FUNCTION_BLOCK FB_IEDClient IMPLEMENTS I_ScsmAbortIndEventSink, I_ScsmGetServerDirectoryCnfEventSink, I_ScsmGetLogicalDeviceDirectoryCnfEventSink, I_ScsmGetLogicalNodeDirectoryCnfEventSink, I_ScsmGetDataValuesCnfEventSink, I_ScsmSetDataValuesCnfEventSink, I_ScsmReportIndEventSink, I_ScsmControlCnfEventSink, I_ScsmLastApplErrorIndEventSink, I_ScsmCommandTerminationIndEventSink,
I_ScsmGetDataSetDirectoryCnfEventSink, I_ScsmCreateDataSetCnfEventSink, I_ScsmDeleteDataSetCnfEventSink
VAR_INPUT
	fbConnection		: FB_iec61850ClientClass := (ipAbortInd:=THIS^, ipGetServerDirectoryCnf:=THIS^, ipGetLogicalDeviceDirectoryCnf:=THIS^, ipGetLogicalNodeDirectoryCnf:=THIS^, ipGetDataValuesCnf:=THIS^, ipSetDataValuesCnf:=THIS^, ipReportInd:=THIS^, ipControlCnf:=THIS^, ipLastApplErrorInd:=THIS^, ipCommandTerminationInd:=THIS^,
													ipGetDataSetDirectoryCnf:=THIS^, ipCreateDataSetCnf:=THIS^, ipDeleteDataSetCnf:=THIS^);
END_VAR
VAR
	_bAbort				: BOOL; (* Rising edge activates AbortReq() command execution *)
	_bDisconnect		: BOOL; (* Rising edge activates ReleaseReq() command execution *)
	_bConnect			: BOOL; (* Rising edge activates AssociateReq() command execution *)
	_bReconnect			: BOOL := TRUE; (* TRUE => reconnect automatically *)
	_bReadAllData		: BOOL := TRUE; (* TRUE => read/refresh all data values on reconnect *)
	
	state				: BYTE;
	eState				: E_AsyncEnvironmentState; (* Environment state *)
	bBusy				: BOOL; (* If TRUE => command execution is busy *)
	bSuccess			: BOOL;
	ipResult			: I_AsyncServiceResultClass;
	sLastErrorResult	: T_MaxString;
	fbAbortReason		: FB_ServiceErrorClass := (stError:=SUCCESS_EVENT);
	sLastAbortReason	: T_MaxString;
	nInvokeID			: UDINT;
	eServiceError		: E_AcsiServiceError; (* Latest OnXyzCnf() or OnXyzInd() event handler error *)
	nServiceError		: UDINT; (* Counts OnXyzCnf() and OnXyzInd() event handler errors *)
	nCmdError			: UDINT; (* Counts xyzReq() command errors *)
	sObjReference		: T_AcsiObjectReference; (* DATA object reference *)
	sCtrlReference		: T_AcsiObjectReference; (* CONTROLLABLE-DATA object reference *)
	
	bGetServerDirectory				: BOOL := TRUE; (* Rising edge enumerates logical-devices *)
	bGetLogicalDeviceDirectory		: BOOL := TRUE; (* Rising edge enumerates logical-nodes *)
	bGetLogicalNodeDirectory		: BOOL := TRUE; (* Rising edge enumerates "IEDLD1/LLN0" data-sets *)
	bGetAllServerValues				: BOOL := TRUE; (* Rising edge reads all "IEDLD1" data attribute values *)
	bGetAllDataValues_LLN0_ST		: BOOL := TRUE; (* Rising edge reads all "IEDLD1/LLN0.ST" data attribute values (having selected functional constraint) *)
	bGetDataValues_LLN0_ST_Beh		: BOOL := TRUE; (* Rising edge reads all "IEDLD1/LLN0.ST.Beh" data attribute values (having selected functional constraint) *)
	
	bCreateDataSet_NonPersistent	: BOOL; (* Rising edge creates non-persistent data-set *)
	bCreateDataSet_Persistent		: BOOL; (* Rising edge creates persistent data-set *)
	
	bDeleteDataSet_NonPersistent	: BOOL; (* Rising edge deletes non-persistent data-set *)
	bDeleteDataSet_Persistent		: BOOL; (* Rising edge deletes persistent data-set *)
	
	bEnable_urcb101_NonPersistent	: BOOL; (* Rising edge enables urcb101 to report non-persistent data-set *)
	bEnable_urcb101_Persistent		: BOOL; (* Rising edge enables urcb101 to report persistent data-set *)
	bEnable_urcb101_DS1				: BOOL; (* Rising edge enables urcb101 to report static data-set *)
	bDisable_urcb101				: BOOL; (* Rising edge disables urcb101 reporting *)
	bSetDataValues_urcb101_DatSet	: BOOL; (* Rising edge writes empty string to "IEDLD1/LLN0.RP.urcb101.DatSet" attribute value *)

	bGetDataSetDirectory_NonPersistent : BOOL;(* Rising edge enumerates member of non-persistent data-set *)
	bGetDataSetDirectory_Persistent	: BOOL;(* Risign edge enumerates member of persistent data-set *)
	bGetDataSetDirectory_DS1		: BOOL;(* Rising edge enumerates member of static data-set *)
	
	(* If non-persistent or persistent data-set is used by any control-block then it is not possible 
		to delete it => Disable reporting and reconfigure the control-block to use an other data-set. *)
	
	fbNonPersistent					: FB_AcsiCommonDataSetClass:=(sObjectName:='NonPersistentDataSet');
	fbPersistent					: FB_AcsiCommonDataSetClass:=(sObjectName:='PersistentDataSet');
END_VAR

fbConnection.Execute();
eState:= fbConnection.eState;

CASE state OF
	0: (* Initial state *)
		IF _bAbort THEN (* Abort connection => execute AbortReq() command *)
			_bAbort:= FALSE;
			bSuccess:= fbConnection.AbortReq(ipReason:=fbAbortReason, ipSink:=0, ipResult=>ipResult);
			state:= SEL(bSuccess, 100, 1);
		ELSIF eState = E_AsyncEnvironmentState.Idle AND (_bConnect OR _bReconnect) THEN (* Open/establish connection => execute AssociateReq() command *)
			_bConnect:= FALSE;
			bGetAllServerValues:= SEL(_bReadAllData, bGetAllServerValues, TRUE);
			bSuccess:= fbConnection.AssociateReq(ipSink:=0, ipResult=>ipResult);
			state:= SEL(bSuccess, 100, 1);
		ELSIF eState = E_AsyncEnvironmentState.Established AND _bDisconnect THEN (* Close/release connection => execute ReleaseReq() command *)
			_bDisconnect:= FALSE;
			bSuccess:= fbConnection.ReleaseReq(ipSink:=0, ipResult=>ipResult);
			state:= SEL(bSuccess, 100, 1);
		ELSIF eState = E_AsyncEnvironmentState.Established THEN (* Connection established => exchange IED data *)
			state:= 10;
		END_IF
		_bConnect:= FALSE;
		_bDisconnect:= FALSE;
		(*==================================================================================================================================================================*)
	1: (* Wait for AbortReq() or ReleaseReq() or AssociateReq() command completion *)
		IF ipResult <> 0 THEN
			ipResult.Execute();
			IF NOT (bBusy:=ipResult.IsBusy()) THEN
				state:= SEL(ipResult.IsCompleted(), 100(* failed or aborted *), 0(* succeeded *));
			END_IF
		END_IF
		(*==================================================================================================================================================================*)
	10: (* Read/Write IED data *)
		IF bGetServerDirectory THEN (* Example => execute GetServerDirectoryReq() command *)
			bGetServerDirectory:= FALSE;
			bSuccess:= fbConnection.GetServerDirectoryReq(ipServer:=fbIED, eClass:=E_AcsiServerDirectoryClass.LogicalDevice, hUser:=0, ipSink:=0, nInvokeID=>nInvokeID, ipResult=>ipResult);
			state:= SEL(bSuccess, 100, 11);
		ELSIF bGetLogicalDeviceDirectory THEN (* Example => execute GetLogicalDeviceDirectoryReq() command *)
			bGetLogicalDeviceDirectory:= FALSE;
			bSuccess:= fbConnection.GetLogicalDeviceDirectoryReq(ipLogicalDevice:=fbIED.IEDLD1, hUser:=0, ipSink:=0, nInvokeID=>nInvokeID, ipResult=>ipResult);
			state:= SEL(bSuccess, 100, 11);
		ELSIF bGetLogicalNodeDirectory THEN (* Example => execute GetLogicalNodeDirectoryReq() command *)
			bGetLogicalNodeDirectory:= FALSE;
			bSuccess:= fbConnection.GetLogicalNodeDirectoryReq(ipLogicalNode:=fbIED.IEDLD1.LLN0, eClass:=E_AcsiLogicalNodeClass.DataSet, hUser:=0, ipSink:=0, nInvokeID=>nInvokeID, ipResult=>ipResult);
			state:= SEL(bSuccess, 100, 11);
		ELSIF bGetAllServerValues THEN (* Example => execute GetAllServerValues() command *)
			bGetAllServerValues:= FALSE;
			bSuccess:= fbConnection.GetAllServerValuesReq(ipServer:=fbIED, hUser:=0, ipSink:=0, nInvokeID=>nInvokeID, ipResult=>ipResult);
			state:= SEL(bSuccess, 100, 11);
		ELSIF bGetAllDataValues_LLN0_ST THEN (* Example => execute GetAllDataValuesReq() command *)
			bGetAllDataValues_LLN0_ST:= FALSE;
			bSuccess:= fbConnection.GetAllDataValuesReq(ipLogicalNode:=fbIED.IEDLD1.LLN0, eFc:=E_AcsiFc.ST_, hUser:=0, ipSink:=0, nInvokeID=>nInvokeID, ipResult=>ipResult);
			state:= SEL(bSuccess, 100, 11);
		ELSIF bGetDataValues_LLN0_ST_Beh THEN (* Example => execute GetDataValuesReq() command *)
			bGetDataValues_LLN0_ST_Beh:= FALSE;
			bSuccess:= fbConnection.GetDataValuesReq(ipData:=fbIED.IEDLD1.LLN0.Beh, eFc:=E_AcsiFc.ST_, hUser:=0, ipSink:=0, nInvokeID=>nInvokeID, ipResult=>ipResult);
			state:= SEL(bSuccess, 100, 11);
		(*==================================================================================================================================================================*)
		ELSIF bCreateDataSet_NonPersistent THEN (* Example => execute CreateDataSet(non-persistent) command *)
			bCreateDataSet_NonPersistent:= FALSE;
			IF fbNonPersistent.nMembers = 0 THEN (* Add some members *)
				bSuccess:= fbNonPersistent.AddMember(ipData:=fbIED.IEDLD1.XCBR1.Pos.stVal, eFc:=E_AcsiFc.ST_);
				bSuccess:= fbNonPersistent.AddMember(ipData:=fbIED.IEDLD1.LLN0.Mod_.stVal, eFc:=E_AcsiFc.ST_);
			END_IF
			bSuccess:= fbConnection.CreateDataSetReq(ipDataSet:=fbNonPersistent, ipLogicalNode:=0(* ipLogicalNode = 0 => non-persistent data-set *), hUser:=0, ipSink:=0, nInvokeID=>nInvokeID, ipResult=>ipResult);
			state:= SEL(bSuccess, 100, 11);
		(*==================================================================================================================================================================*)
		ELSIF bCreateDataSet_Persistent THEN (* Example => execute CreateDataSet(persistent) command *)
			bCreateDataSet_Persistent:= FALSE;
			IF fbPersistent.nMembers = 0 THEN (* Add some members *)
				bSuccess:= fbPersistent.AddMember(ipData:=fbIED.IEDLD1.MMXU1.TotW.mag.f, eFc:=E_AcsiFc.MX);
				bSuccess:= fbPersistent.AddMember(ipData:=fbIED.IEDLD1.LLN0.Beh.stVal, eFc:=E_AcsiFc.ST_);
			END_IF
			bSuccess:= fbConnection.CreateDataSetReq(ipDataSet:=fbPersistent, ipLogicalNode:=fbIED.IEDLD1.LLN0 (* ipLogicalNode <> 0 => persistent data-set *), hUser:=0, ipSink:=0, nInvokeID=>nInvokeID, ipResult=>ipResult);
			state:= SEL(bSuccess, 100, 11);
		(*==================================================================================================================================================================*)
		ELSIF bDeleteDataSet_NonPersistent THEN (* Example => execute DeleteDataSet(non-persistent) command *)
			bDeleteDataSet_NonPersistent:= FALSE;
			bSuccess:= fbConnection.DeleteDataSetReq(ipDataSet:=fbNonPersistent, hUser:=0, ipSink:=0, nInvokeID=>nInvokeID, ipResult=>ipResult);
			state:= SEL(bSuccess, 100, 11);
		(*==================================================================================================================================================================*)
		ELSIF bDeleteDataSet_Persistent THEN (* Example => execute DeleteDataSet(persistent) command *)
			bDeleteDataSEt_Persistent:= FALSE;
			bSuccess:= fbConnection.DeleteDataSetReq(ipDataSet:=fbPersistent, hUser:=0, ipSink:=0, nInvokeID=>nInvokeID, ipResult=>ipResult);
			state:= SEL(bSuccess, 100, 11);
		(*==================================================================================================================================================================*)
		ELSIF bEnable_urcb101_NonPersistent THEN (* Example => Enable urcb101 to use dynamic created non-persistent data-set *)
			bEnable_urcb101_NonPersistent:= FALSE;
			bSuccess:= fbIED.IEDLD1.LLN0.urcb101.Client.EnableReq(ipClient:=fbConnection, ipDataSet:=fbNonPersistent, ipResult=>ipResult);
			state:= SEL(bSuccess, 100, 11);
		(*==================================================================================================================================================================*)
		ELSIF bEnable_urcb101_Persistent THEN (* Example => Enable urcb101 to use dynamic created persistent data-set *)
			bEnable_urcb101_Persistent:= FALSE;
			bSuccess:= fbIED.IEDLD1.LLN0.urcb101.Client.EnableReq(ipClient:=fbConnection, ipDataSet:=fbPersistent, ipResult=>ipResult);
			state:= SEL(bSuccess, 100, 11);
		(*==================================================================================================================================================================*)
		ELSIF bEnable_urcb101_DS1 THEN (* Example => Enable urcb101 to use static data-set *)
			bEnable_urcb101_DS1:= FALSE;
			bSuccess:= fbIED.IEDLD1.LLN0.urcb101.Client.EnableReq(ipClient:=fbConnection, ipDataSet:=fbIED.IEDLD1.LLN0.DS1, ipResult=>ipResult);
			state:= SEL(bSuccess, 100, 11);
		(*==================================================================================================================================================================*)
		ELSIF bDisable_urcb101 THEN (* Example => Disable urcb101 *)
			bDisable_urcb101:= FALSE;
			bSuccess:= fbIED.IEDLD1.LLN0.urcb101.Client.DisableReq(ipResult=>ipResult);
			state:= SEL(bSuccess, 100, 11);
		(*==================================================================================================================================================================*)
		ELSIF bSetDataValues_urcb101_DatSet THEN(* Example => Set "DatSet" attribute value to empty string *)
			bSetDataValues_urcb101_DatSet:= FALSE;
			fbIED.IEDLD1.LLN0.urcb101.DatSet.sValue:= '';(* Set local "DatSet" attribute value to empty string *)
			(* Activate method to set the remote "DatSet" attribute value to empty string *)
			bSuccess:= fbConnection.SetDataValuesReq(ipData:=fbIED.IEDLD1.LLN0.urcb101.DatSet, eFc:=E_AcsiFc.RP, hUser:=0, ipSink:=0, nInvokeID=>nInvokeID, ipResult=>ipResult);
			state:= SEL(bSuccess, 100, 11);
		(*==================================================================================================================================================================*)
		ELSIF bGetDataSetDirectory_NonPersistent THEN (* Example => Enumerate member of non-persistent data-set *)
			bGetDataSetDirectory_NonPersistent:= FALSE;
			bSuccess:= fbConnection.GetDataSetDirectoryReq(ipDataSet:=fbNonPersistent, hUser:=0, ipSink:=0, nInvokeID=>nInvokeID, ipResult=>ipResult);
			state:= SEL(bSuccess, 100, 11);
		(*==================================================================================================================================================================*)
		ELSIF bGetDataSetDirectory_Persistent THEN (* Example => Enumerate member of persistent data-set *)
			bGetDataSetDirectory_Persistent:= FALSE;
			bSuccess:= fbConnection.GetDataSetDirectoryReq(ipDataSet:=fbPersistent, hUser:=0, ipSink:=0, nInvokeID=>nInvokeID, ipResult=>ipResult);
			state:= SEL(bSuccess, 100, 11);
		(*==================================================================================================================================================================*)
		ELSIF bGetDataSetDirectory_DS1 THEN (* Example => Enumerate member of static data-set *)
			bGetDataSetDirectory_DS1:= FALSE;
			bSuccess:= fbConnection.GetDataSetDirectoryReq(ipDataSet:=fbIED.IEDLD1.LLN0.DS1, hUser:=0, ipSink:=0, nInvokeID=>nInvokeID, ipResult=>ipResult);
			state:= SEL(bSuccess, 100, 11);
		ELSE
			state:= 0;
		END_IF
		(*==================================================================================================================================================================*)
	11: (* Wait for GetServerDirectoryReq(), GetLogicalDeviceDirectoryReq(), GetLogicalNodeDirectoryReq(), GetAllServerValuesReq(), GetAllDataValuesReq() or GetDataValuesReq() command completion *)
		IF ipResult <> 0 THEN
			ipResult.Execute();
			IF NOT (bBusy:=ipResult.IsBusy()) THEN
				state:= SEL(ipResult.IsCompleted(), 100(* failed or aborted *), 0(* succeeded *));
			END_IF
		END_IF
		(*==================================================================================================================================================================*)
	100: (* Error state *)
		state:= 0;
		IF ipResult <> 0 THEN
			nCmdError:= nCmdError + 1;
			sLastErrorResult:= ipResult.Dump();
		END_IF
END_CASE

PROPERTY bAbort : BOOL
SET
_bAbort:= bAbort;
END_SET
END_PROPERTY

PROPERTY bConnect : BOOL
SET
_bConnect:= bConnect;
END_SET
END_PROPERTY

PROPERTY bDisconnect : BOOL
SET
_bDisconnect:= bDisconnect;
END_SET
END_PROPERTY

PROPERTY bReconnect : BOOL
SET
_bReconnect:= bReconnect;
END_SET
END_PROPERTY

(* This method receives IEC61850::Abort.ind primitive. *)
METHOD OnAbortInd
VAR_INPUT
	ipAA		: I_ScsmAssociationClass; (* Application association. If = 0 => optional. *)
	bPAbort		: BOOL; (* TRUE => P-Abort.request(), issued by provider, FALSE => Abort.request(), issued by user. *)
	ipReason	: I_ServiceErrorClass; (* Abort reason. *)
	ipData		: I_BaseStreamClass; (* Optional data. If = 0 => default, no data. *)
END_VAR
VAR
END_VAR
IF ipReason <> 0 THEN
	sLastAbortReason:= ipReason.Dump();
END_IF
END_METHOD

(* This method receives buffered IEC61850::Report.ind primitive. *)
METHOD OnBufferedReportInd
VAR_INPUT
	ipAA		: I_ScsmAssociationClass; (* Application association. If = 0 => optional. *)
	info		: ST_ScsmReportEventInfo;
	ipBrcb		: I_AcsiCommonBufferedReportControlBlockClass; (* Interface pointer to BRCB object. *)
	ipDataSet	: I_AcsiCommonDataSetClass; (* Interface pointer to data-set object. *)
	ipData		: I_AcsiCommonDataClass; (* Interface pointer to reported data object. *)
	eFc			: E_AcsiFc; (* Functional constraint of reported data. *)
	eError		: E_AcsiServiceError; (* Data access error code. *)
END_VAR
VAR
END_VAR
IF eError <> E_AcsiServiceError.NoError THEN
	eServiceError:= eError;
	nServiceError:= nServiceError + 1;
END_IF
IF ipData <> 0 THEN
	sObjReference:= ipData.GetObjectReference();
END_IF
END_METHOD

(* This method receives IEC61850::CommandTermination.ind primitive. *)
METHOD OnCommandTerminationInd
VAR_INPUT
	ipAA		: I_ScsmAssociationClass; (* Application association. If = 0 => optional. *)
	info		: ST_ScsmCommandTerminationEventInfo;
	ipCtrl		: I_AcsiCommonControllableDataClass; (* Interface pointer to controllable data object. *)
	ipData		: I_AcsiCommonDataClass; (* Interface pointer to Oper/Cancel/SBO or SBOw data object. *)
	eFc			: E_AcsiFc; (* Functional constraint (CO). *)
	eError		: E_AcsiServiceError; (* Error code. *)
END_VAR
VAR
END_VAR
IF eError <> E_AcsiServiceError.NoError THEN
	eServiceError:= eError;
	nServiceError:= nServiceError + 1;
END_IF
IF ipCtrl <> 0 THEN
	sCtrlReference:= ipCtrl.GetObjectReference();
END_IF
IF ipData <> 0 THEN
	sObjReference:= ipData.GetObjectReference();
END_IF
END_METHOD

(* This method receives IEC61850::Control[Select|Operate|SelectWithValue|Cancel].cnf primitive. *)
METHOD OnControlCnf
VAR_INPUT
	ipAA		: I_ScsmAssociationClass; (* Application association. If = 0 => optional. *)
	info		: ST_ScsmConfirmedEventInfo;
	ipCtrl		: I_AcsiCommonControllableDataClass; (* Interface pointer to controllable data object. *)
	ipData		: I_AcsiCommonDataClass; (* Interface pointer to Oper/Cancel/SBO or SBOw data object. *)
	eFc			: E_AcsiFc; (* Functional constraint (CO). *)
	eError		: E_AcsiServiceError; (* Write/Read data access error code. *)
END_VAR
VAR
END_VAR
IF eError <> E_AcsiServiceError.NoError THEN
	eServiceError:= eError;
	nServiceError:= nServiceError + 1;
END_IF
IF ipCtrl <> 0 THEN
	sCtrlReference:= ipCtrl.GetObjectReference();
END_IF
IF ipData <> 0 THEN
	sObjReference:= ipData.GetObjectReference();
END_IF
END_METHOD

(* This method receives Scsm::CreateDataSet.cnf primitive. *)
METHOD OnCreateDataSetCnf
VAR_INPUT
	ipAA		: I_ScsmAssociationClass; (* Application association. If = 0 => optional. *)
	info		: ST_ScsmConfirmedEventInfo;
	ipDataSet	: I_AcsiCommonDataSetClass; (* Data-set to be created *)
	eError		: E_AcsiServiceError; (* Data-set access error code. *)
END_VAR
IF eError <> E_AcsiServiceError.NoError THEN
	eServiceError:= eError;
	nServiceError:= nServiceError + 1;
END_IF
IF ipDataSet <> 0 THEN
	sObjReference:= ipDataSet.GetObjectReference();
END_IF
END_METHOD

(* This method receives Scsm::DeleteDataSet.cnf primitive. *)
METHOD OnDeleteDataSetCnf
VAR_INPUT
	ipAA		: I_ScsmAssociationClass; (* Application association. If = 0 => optional. *)
	info		: ST_ScsmConfirmedEventInfo;
	ipDataSet	: I_AcsiCommonDataSetClass; (* Data-set to be deleted *)
	eError		: E_AcsiServiceError; (* Data-set access error code. *)
END_VAR
IF eError <> E_AcsiServiceError.NoError THEN
	eServiceError:= eError;
	nServiceError:= nServiceError + 1;
END_IF
IF ipDataSet <> 0 THEN
	sObjReference:= ipDataSet.GetObjectReference();
END_IF
END_METHOD

(* This method receives Scsm::GetDataSetDirectory.cnf primitive. *)
METHOD OnGetDataSetDirectoryCnf
VAR_INPUT
	ipAA				: I_ScsmAssociationClass; (* Application association. If = 0 => optional. *)
	info				: ST_ScsmConfirmedEventInfo;
	ipDataSet			: I_AcsiCommonDataSetClass; (* Interface pointer to data-set object. *)
	sObjectReference	: T_AcsiObjectReference; (* Data-set member object reference. *)
	eFc					: E_AcsiFc; (* Data-set member functional constraint. *)
	eError				: E_AcsiServiceError; (* Data-set member access error code. *)
END_VAR
IF eError <> E_AcsiServiceError.NoError THEN
	eServiceError:= eError;
	nServiceError:= nServiceError + 1;
END_IF
sObjReference:= sObjectReference;
END_METHOD

(* This method receives IEC61850::GetDataValues.cnf primitive. *)
METHOD OnGetDataValuesCnf
VAR_INPUT
	ipAA		: I_ScsmAssociationClass; (* Application association. If = 0 => optional. *)
	info		: ST_ScsmConfirmedEventInfo;
	ipData		: I_AcsiCommonDataClass; (* Interface pointer to read data object. *)
	eFc			: E_AcsiFc; (* Functional constraint of read data. *)
	eError		: E_AcsiServiceError; (* Data access error code. *)
END_VAR
VAR
END_VAR
IF eError <> E_AcsiServiceError.NoError THEN
	eServiceError:= eError;
	nServiceError:= nServiceError + 1;
END_IF
IF ipData <> 0 THEN
	sObjReference:= ipData.GetObjectReference();
END_IF
END_METHOD

(* This method receives IEC61850::GetLogicalDeviceDirectory.cnf primitive. *)
METHOD OnGetLogicalDeviceDirectoryCnf
VAR_INPUT
	ipAA				: I_ScsmAssociationClass; (* Application association. If = 0 => optional. *)
	info				: ST_ScsmConfirmedEventInfo;
	ipLogicalDevice		: I_AcsiCommonLogicalDeviceClass; (* Interface pointer to logical-device object. *)
	sObjectReference	: T_AcsiObjectReference;
	eError				: E_AcsiServiceError; (* Logical-device class access error code. *)
END_VAR
VAR
END_VAR
IF eError <> E_AcsiServiceError.NoError THEN
	eServiceError:= eError;
	nServiceError:= nServiceError + 1;
END_IF
sObjReference:= sObjectReference;
END_METHOD

(* This method receives IEC61850::GetLogicalNodeDirectory.cnf primitive. *)
METHOD OnGetLogicalNodeDirectoryCnf
VAR_INPUT
	ipAA				: I_ScsmAssociationClass; (* Application association. If = 0 => optional. *)
	info				: ST_ScsmConfirmedEventInfo;
	ipLogicalNode		: I_AcsiCommonLogicalNodeClass; (* Interface pointer to logical-node object. *)
	eClass				: E_AcsiLogicalNodeClass; (* Logical-node directory class (BRCB, URCB, DATA-SET, ... ). *)
	sObjectReference	: T_AcsiObjectReference;
	eError				: E_AcsiServiceError; (* Logical-node class access error code. *)
END_VAR
VAR
END_VAR
IF eError <> E_AcsiServiceError.NoError THEN
	eServiceError:= eError;
	nServiceError:= nServiceError + 1;
END_IF
sObjReference:= sObjectReference;
END_METHOD

(* This method receives IEC61850::GetServerDirectory.cnf primitive. *)
METHOD OnGetServerDirectoryCnf
VAR_INPUT
	ipAA				: I_ScsmAssociationClass; (* Application association. If = 0 => optional. *)
	info				: ST_ScsmConfirmedEventInfo;
	ipServer			: I_AcsiCommonIntelligentElectronicDeviceClass; (* Interface pointer to server object. *)
	eClass				: E_AcsiServerDirectoryClass; (* Server directory class (logical-device or file). *)
	sObjectReference	: T_AcsiObjectReference;
	eError				: E_AcsiServiceError; (* Server class (logical-device) access error code. *)
END_VAR
VAR
END_VAR
IF eError <> E_AcsiServiceError.NoError THEN
	eServiceError:= eError;
	nServiceError:= nServiceError + 1;
END_IF
sObjReference:= sObjectReference;
END_METHOD

(* This method receives IEC61850::LastApplError.ind primitive. *)
METHOD OnLastApplErrorInd
VAR_INPUT
	ipAA		: I_ScsmAssociationClass; (* Application association. If = 0 => optional. *)
	info		: ST_ScsmAdditionalCauseDiagnosticEventInfo;
	ipCtrl		: I_AcsiCommonControllableDataClass; (* Interface pointer to controllable data object. *)
	eError		: E_AcsiServiceError; (* Error code. *)
END_VAR
VAR
END_VAR
IF eError <> E_AcsiServiceError.NoError THEN
	eServiceError:= eError;
	nServiceError:= nServiceError + 1;
END_IF
IF ipCtrl <> 0 THEN
	sCtrlReference:= ipCtrl.GetObjectReference();
END_IF
END_METHOD

(* This method receives IEC61850::SetDataValues.cnf primitive. *)
METHOD OnSetDataValuesCnf
VAR_INPUT
	ipAA		: I_ScsmAssociationClass; (* Application association. If = 0 => optional. *)
	info		: ST_ScsmConfirmedEventInfo;
	ipData		: I_AcsiCommonDataClass; (* Interface pointer to written data object. *)
	eFc			: E_AcsiFc; (* Functional constraint of written data. *)
	eError		: E_AcsiServiceError; (* Data access error code. *)
END_VAR
VAR
END_VAR
IF eError <> E_AcsiServiceError.NoError THEN
	eServiceError:= eError;
	nServiceError:= nServiceError + 1;
END_IF
IF ipData <> 0 THEN
	sObjReference:= ipData.GetObjectReference();
END_IF
END_METHOD

(* This method receives unbuffered IEC61850::Report.ind primitive. *)
METHOD OnUnbufferedReportInd
VAR_INPUT
	ipAA		: I_ScsmAssociationClass; (* Application association. If = 0 => optional. *)
	info		: ST_ScsmReportEventInfo;
	ipUrcb		: I_AcsiCommonUnbufferedReportControlBlockClass; (* Interface pointer to URCB object. *)
	ipDataSet	: I_AcsiCommonDataSetClass; (* Interface pointer to dataset object. *)
	ipData		: I_AcsiCommonDataClass; (* Interface pointer to reported data object. *)
	eFc			: E_AcsiFc; (* Functional constraint of reported data. *)
	eError		: E_AcsiServiceError; (* Data access error code. *)
END_VAR
VAR
END_VAR
IF eError <> E_AcsiServiceError.NoError THEN
	eServiceError:= eError;
	nServiceError:= nServiceError + 1;
END_IF
IF ipData <> 0 THEN
	sObjReference:= ipData.GetObjectReference();
END_IF
END_METHOD

END_FUNCTION_BLOCK
